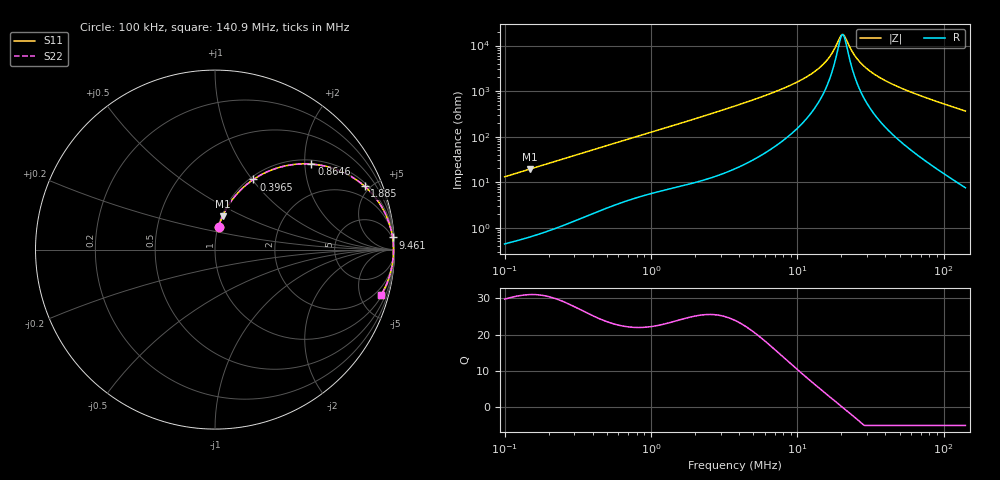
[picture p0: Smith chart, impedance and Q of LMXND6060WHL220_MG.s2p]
! LMXND6060WHL220_MG  S-PARAMETER MODEL  ( General Type )
! Model Generated by TAIYO YUDEN Corporation (http://www.ty-top.com)
! Version 1.0
! TAIYO YUDEN Control No. 191025NI43SB-FBB
! Copyright(c) 2019 TAIYO YUDEN CO.,LTD. All Rights Reserved.
! Product Description (link to TY-COMPAS)
! https://ds.yuden.co.jp/TYCOMPAS/or/detail?pn=LMXND6060WHL220MMG&u=M
! Products Name : Inductors
! Characteristics :
!  Inductance : 22 uH , SRF(min) : 12 MHz , DC Resistance(max) : 0.1755 Ohm
!  Rated Current : Saturation :1300 mA , Temp Rise : 1400 mA
!  Case Size : 6.0 x 6.0 / 0.236 x 0.236 [mm/inch] , Thickness : 2.8 / 0.11 [mm/inch]
!  (Conditions: Temperature = 25 degC , DC Bias Current/Voltage = 0A / 0V)
! External Node Assignments :
!  1  o---GGG---o  2
! GND o---------o GND
! Frequency Range : 0.1MHz  -  140.89697MHz  [ 402 STEP ]
# MHz S RI R 50
! Freq[MHz].  S11 Real  S11 Imag  S21 Real  S21 Imag  S12 Real  S12 Imag  S22 Real  S22 Imag
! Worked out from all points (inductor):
!   401 points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, 100 kHz to 140.9 MHz, reference 50 ohm
!   read as one part in series: L = 20.8 uH near 103.7 kHz
!   highest Q = 31 at 149 kHz (marker M1), where L = 20.7 uH
!   self-resonance near 20.26 MHz
!   S11 on the Smith chart (normalised r, x): 100 kHz: 1.01, +0.26; 396.5 kHz: 1.04, +1.02; 864.6 kHz: 1.10, +2.16; 1.885 MHz: 1.19, +4.64; 9.461 MHz: 4, +29; 140.9 MHz: 1.15, -7.30
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0.1  0.021 0.1276  0.979 -0.1276  0.979 -0.1276  0.021 0.1276
0.149001  0.0419 0.1848  0.9581 -0.1848  0.9581 -0.1848  0.0419 0.1848
0.336853  0.1673 0.3549  0.8327 -0.3549  0.8327 -0.3549  0.1673 0.3549
0.396544  0.2145 0.3912  0.7855 -0.3912  0.7855 -0.3912  0.2145 0.3912
0.601663  0.3728 0.4619  0.6272 -0.4619  0.6272 -0.4619  0.3728 0.4619
0.864566  0.5375 0.4764  0.4625 -0.4764  0.4625 -0.4764  0.5375 0.4764
1.134703  0.6582 0.4527  0.3418 -0.4527  0.3418 -0.4527  0.6582 0.4527
1.884973  0.8339 0.3527  0.1661 -0.3527  0.1661 -0.3527  0.8339 0.3527
3.753625  0.9492 0.1996  0.0508 -0.1996  0.0508 -0.1996  0.9492 0.1996
9.460973  0.9893 0.0674  0.0107 -0.0674  0.0107 -0.0674  0.9893 0.0674
12.64421  0.9926 0.0397  0.00741 -0.0397  0.00741 -0.0397  0.9926 0.0397
16.0041  0.9939 0.0197  0.0061 -0.0197  0.0061 -0.0197  0.9939 0.0197
17.52235  0.9942 0.0123  0.00583 -0.0123  0.00583 -0.0123  0.9942 0.0123
19.53556  0.9943 0.0035  0.00566 -0.0035  0.00566 -0.0035  0.9943 0.0035
20.62732  0.9944 -0.000858  0.00564 0.000858  0.00564 0.000858  0.9944 -0.000858
21.38884  0.9944 -0.00376  0.00564 0.00376  0.00564 0.00376  0.9944 -0.00376
24.28248  0.9942 -0.014  0.0058 0.014  0.0058 0.014  0.9942 -0.014
27.56759  0.9938 -0.0244  0.00619 0.0244  0.00619 0.0244  0.9938 -0.0244
33.04618  0.9928 -0.0401  0.00719 0.0401  0.00719 0.0401  0.9928 -0.0401
42.59248  0.9903 -0.0642  0.00971 0.0642  0.00971 0.0642  0.9903 -0.0642
70.75481  0.9784 -0.1253  0.0216 0.1253  0.0216 0.1253  0.9784 -0.1253
140.897  0.9257 -0.2521  0.0743 0.2521  0.0743 0.2521  0.9257 -0.2521
